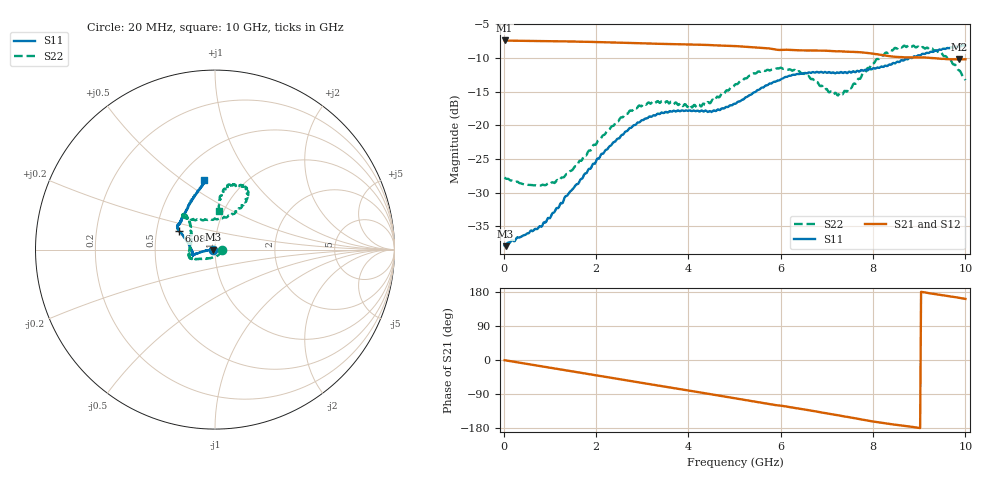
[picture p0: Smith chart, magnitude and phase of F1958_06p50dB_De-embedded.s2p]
! Integrated Device Technology
! Corporate Headquarters
! 6024 Silver Creek Valley Road
! San Jose, CA 95138  USA
! Phone:  1-408-284-8200
! Toll Free:  1-800-223-1366
! Webpage:  http://www.idt.com/
! Timing and RF Division
! 515 Groton Road, Suite 102
! Westford, MA 01886-6024
! Device:  F1958
! Description: 7-bit 0.25 dB Digital Step Attenuator
! Frequency:  0.001 -  6.000 GHz
! Package:  4x4 mm Thin QFN Plastic Package: 24 pin
! Ports:  2 RF, 12 DC
!  Pin  1  = D0
!  Pin  2  = VDD
!  Pin  3  = VMODE
!  Pin  4  = GND
!  Pin  5  = RF1  =  Port 1
!  Pin  6  = GND
!  Pin  7  = GND
!  Pin  8  = GND
!  Pin  9  = GND
!  Pin 10  = GND
!  Pin 11  = GND
!  Pin 12  = GND
!  Pin 13  = GND
!  Pin 14  = RF2  =  Port 2
!  Pin 15  = GND
!  Pin 16  = LE
!  Pin 17  = CLK
!  Pin 18  = DATA
!  Pin 19  = D6
!  Pin 20  = D5
!  Pin 21  = D4
!  Pin 22  = D3
!  Pin 23  = D2
!  Pin 24  = D1
! State:  26
! Atten State:  6.50 dB
! Voltage:  +3.30 Volts
! Current:  0.258 mA
! Data:  The device was measured on a F1958 evaluation board which has
!  individual transmission lines to the RF pins.  Data was collected
!  using a calibrated network analyzer.  The evaluation board was
!  de-embedded using Automatic Fixture Removal (AFR).
!  The reference plane is the edge of the package pin.
! Misc:
!  Action Tracker AT0419
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# GHz S dB R 50
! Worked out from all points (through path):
!   500 points, 20 MHz to 10 GHz, reference 50 ohm
!   highest |S21| = -7.42 dB at 20 MHz (marker M1); lowest = -10.2 dB at 9.86 GHz (marker M2)
!   group delay of S21, straight-line fit = 55.5 ps
!   lowest |S11| = -37.9 dB at 40 MHz (marker M3), VSWR 1.03, Z = 48.7 - j0.0966 ohm
!   |S11| at or under -10 dB: start of sweep to 8.79 GHz; 8.814601 GHz to 8.849401 GHz (34.8 MHz wide, 0.394 % of centre)
!   |S22| runs from -28.9 to -8.1 dB; largest |S21 - S12| = 0.0014
!   S11 on the Smith chart (normalised r, x): 20 MHz: 0.97, -0.00; 6.08 GHz: 0.65, +0.14; 10 GHz: 0.67, +0.61
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0.02  -37.84 -176.2  -7.42 -0.5  -7.42 -0.5  -27.73 -3.8
0.04  -37.92 -175.5  -7.43 -1.0  -7.43 -0.9  -27.87 -5.9
0.44  -36.30 175.0  -7.49 -9.0  -7.49 -9.0  -28.79 -26.1
0.96  -33.74 -179.3  -7.52 -19.5  -7.52 -19.5  -28.66 -62.8
1.3  -31.11 -176.1  -7.56 -26.3  -7.55 -26.3  -27.72 -92.3
1.7  -27.90 -173.0  -7.61 -34.3  -7.60 -34.3  -25.11 -121.9
2.62  -21.06 -169.1  -7.77 -52.8  -7.76 -52.8  -18.41 -154.0
3.36  -18.32 -165.8  -7.92 -67.7  -7.92 -67.8  -16.57 -163.4
4.24  -17.97 -169.8  -8.06 -85.3  -8.07 -85.3  -16.97 165.7
5.02  -16.80 170.7  -8.26 -101.2  -8.27 -101.2  -13.91 134.3
5.52  -14.75 159.1  -8.49 -111.3  -8.50 -111.3  -12.01 130.5
6.08  -12.91 152.5  -8.81 -121.9  -8.82 -121.9  -11.61 132.6
6.68  -12.15 148.1  -8.91 -133.9  -8.93 -133.8  -13.13 128.5
7.08  -12.23 145.2  -8.99 -142.8  -9.00 -142.6  -14.98 108.1
7.3  -12.11 143.1  -9.04 -147.1  -9.05 -147.0  -15.24 90.3
7.9  -11.75 132.3  -9.30 -160.2  -9.29 -160.2  -11.50 60.2
8.34  -11.03 122.6  -9.74 -168.6  -9.74 -168.7  -9.12 58.3
8.76  -10.19 112.9  -9.94 -175.0  -9.95 -175.0  -8.17 64.7
9.26  -9.09 104.2  -10.03 175.4  -10.03 175.4  -8.61 76.8
9.54  -8.65 101.1  -10.15 170.2  -10.18 170.2  -9.76 81.6
9.86  -8.28 98.8  -10.24 164.3  -10.28 164.4  -11.84 83.9
10  -8.17 98.9  -10.21 161.2  -10.24 161.3  -13.31 83.5
